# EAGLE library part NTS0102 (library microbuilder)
NTS0102 - I2C Level Shifter The NTS0102 is a 2-bit, open-drain, dual supply translating transceiver with auto direction sensing, that enables bidirectional voltage level translation. VCCA: 1.65-3.6V VCCB: 2.3V-5.5V Max Data Rate: 50 Mbps Temperature: -40°C - 125°C XSON8 Package (NTS0102GT) - Mouser: 771-NTS0102GT115
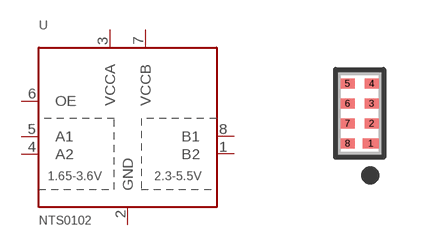
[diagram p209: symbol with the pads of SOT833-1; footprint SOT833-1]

Designator prefix U

## NTS0102XSON8  [SOT833-1]
1  B2
2  GND
3  VCCA
4  A2
5  A1
6  OE
7  VCCB
8  B1

## Footprint SOT833-1 (pad centres in mm)
Source: http://ics.nxp.com/packaging/package.outlines/pdf/sot833-1.pdf
smd 0.4 x 0.25: 1 0.275,-0.75
smd 0.35 x 0.25: 2 0.3,-0.25; 3 0.3,0.25; 4 0.3,0.75; 5 -0.3,0.75; 6 -0.3,0.25; 7 -0.3,-0.25; 8 -0.3,-0.75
